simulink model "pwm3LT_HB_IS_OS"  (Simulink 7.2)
settings: Solver=ode3  SolverMode=SingleTasking  StartTime=0.0  StopTime=0.1  FixedStep=10e-6  MaxStep=1e-4  RelTol=1e-3
libraries: PE_CONV_OS x1

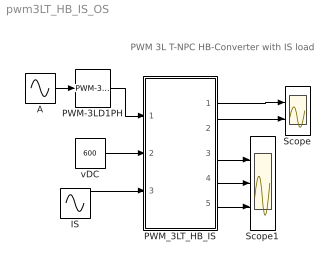
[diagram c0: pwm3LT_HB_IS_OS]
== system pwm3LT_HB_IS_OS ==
  note: PWM 3L T-NPC HB-Converter with IS load
  A : Sin  Amplitude=.8  Frequency=2*pi*50  Phase=[0 ]  SampleTime=0
  IS : Sin  Amplitude=400  Frequency=2*pi*50  Phase=[0 ]  SampleTime=0
  PWM-3LD1PH : PE_CONV_OS/Converter_Control/PWM-3LD1PH  SystemSampleTime=-1  FT=900  PHT=0  A=0.5  O1=0.5  O2=-0.5  DT=1e-6
  PWM_3LT_HB_IS : Subsystem
  Scope : Scope  NumInputPorts=2
  Scope1 : Scope  NumInputPorts=3
  vDC : Constant  Value=600  OutDataType=sfix(16)  OutScaling=2^0
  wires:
  A/1 -> PWM-3LD1PH/1
  PWM_3LT_HB_IS/3("iT1, iD1,vT1") -> Scope1/1
  PWM_3LT_HB_IS/4("iT2, iD2,vT2") -> Scope1/2
  PWM_3LT_HB_IS/5(iDC1,iDC2) -> Scope1/3
  PWM_3LT_HB_IS/1(vA) -> Scope/1
  IS/1 -> PWM_3LT_HB_IS/3(iS)
  vDC/1 -> PWM_3LT_HB_IS/2(vDC)
  PWM-3LD1PH/1 -> PWM_3LT_HB_IS/1(Sw)
  PWM_3LT_HB_IS/2(iA) -> Scope/2

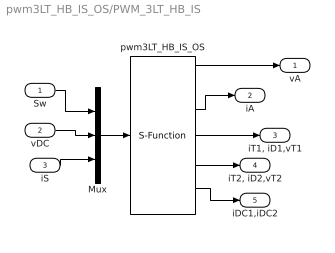
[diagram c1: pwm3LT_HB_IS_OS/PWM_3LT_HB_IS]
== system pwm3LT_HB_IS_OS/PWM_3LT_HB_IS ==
  Sw : Inport  OutDataType=sfix(16)  OutScaling=2^0
  vDC : Inport  Port=2  OutDataType=sfix(16)  OutScaling=2^0
  iS : Inport  Port=3  OutDataType=sfix(16)  OutScaling=2^0
  Mux : Mux  Inputs="[4  1  1]"
  pwm3LT_HB_IS_OS : S-Function  FunctionName=s_pwm_3LT_HB_IS_OS  Parameters=0  EnableBusSupport=off
  vA : Outport  OutDataType=sfix(16)  OutScaling=2^0
  iA : Outport  Port=2  OutDataType=sfix(16)  OutScaling=2^0
  "iT1, iD1,vT1" : Outport  Port=3  OutDataType=sfix(16)  OutScaling=2^0
  "iT2, iD2,vT2" : Outport  Port=4  OutDataType=sfix(16)  OutScaling=2^0
  iDC1,iDC2 : Outport  Port=5  OutDataType=sfix(16)  OutScaling=2^0
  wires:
  pwm3LT_HB_IS_OS/1 -> vA/1
  iS/1 -> Mux/3
  Mux/1 -> pwm3LT_HB_IS_OS/1
  vDC/1 -> Mux/2
  Sw/1 -> Mux/1
  pwm3LT_HB_IS_OS/2 -> iA/1
  pwm3LT_HB_IS_OS/3 -> "iT1, iD1,vT1"/1
  pwm3LT_HB_IS_OS/4 -> "iT2, iD2,vT2"/1
  pwm3LT_HB_IS_OS/5 -> iDC1,iDC2/1
